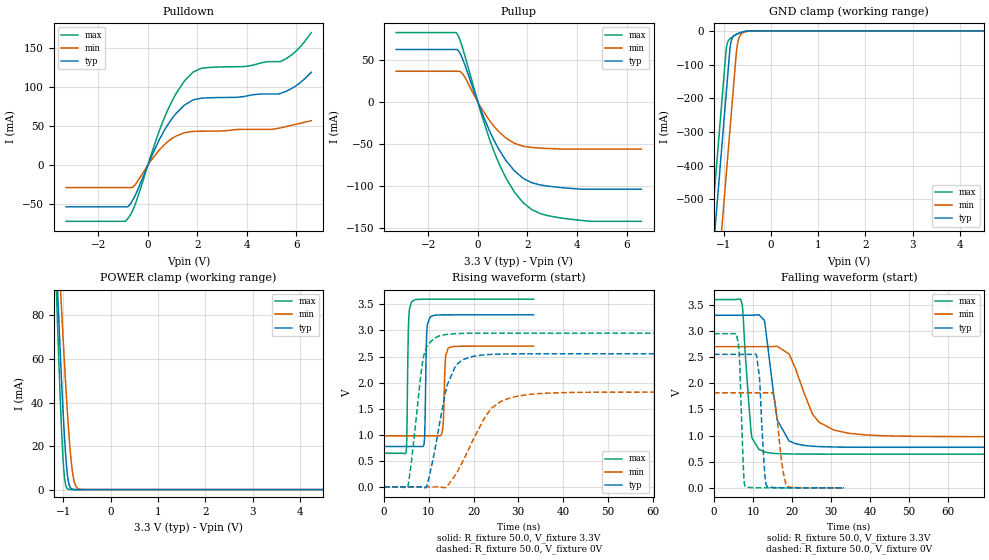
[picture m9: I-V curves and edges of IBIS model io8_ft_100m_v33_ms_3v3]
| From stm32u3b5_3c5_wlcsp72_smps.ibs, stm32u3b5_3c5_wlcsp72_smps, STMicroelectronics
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[Model]   io8_ft_100m_v33_ms_3v3
Model_type I/O
Polarity   Non-Inverting
Enable   Active-Low
| CAP_THRESHOLD on pad IOFT is "UDTCAPC" :
| Rising=30.0% of vddiom   Falling=70.0% of vddiom
| C_comp min and max val. don't necessarily correlate with the min and max pvt
| but are the smallest and greatest pad capacitance found.
| var   typ   min   max
C_comp   5.13864pF  4.98765pF  5.13964pF
|C_comp_pullup   3.32248pF  3.08554pF  3.41453pF
|C_comp_pulldown   1.81616pF  1.90210pF  1.72511pF
Vinl = 1.35V
Vinh = 1.8V
Vmeas = 1.65V   | Reference voltage for timing measurements
Cref  = 50.0pF   | Timing specification test load capacitance value
Rref  = 1.0MOhm   | Timing specification test load resistance value
Vref  = 1.815V   | Timing specification test load voltage
[Model Spec]
| TIME_THRESHOLD on pin ZIV33M is "CMOS" :
| Rising=50.0% of vddiom   Falling=50.0% of vddiom
Vinl 1.27350V 1.06350V 1.35850V
Vinh 1.78850V 1.51250V 1.89250V
| variable   typ   min   max
[Temperature Range] 25.0 130.0 -40.0
| variable   typ   min   max
[Voltage Range] 3.3V 2.7V 3.6V
| variable   typ   min   max
[POWER Clamp Reference] 3.3V 2.7V 3.6V
| variable   typ   min   max
[GND Clamp Reference] 0V 0V 0V
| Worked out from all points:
|   slope of the pulldown table from 0 to 0.495 V, typ, clamps not added: 14.3 ohm
|   slope of the pullup table from 0 to 0.495 V, typ, clamps not added: 13.8 ohm
|   GND clamp passes 1 mA (typ) near -0.50 V on its own axis
|   POWER clamp passes 1 mA (typ) near -0.85 V on its own axis
|   rising waveform, R_fixture 50.0, V_fixture 3.3V: 20-80 % time 305ps typ, 372ps min, 294ps max; typ from 0.776 V to 3.3 V
|   falling waveform, R_fixture 50.0, V_fixture 3.3V: 20-80 % time 2.69ns typ, 5.74ns min, 1.65ns max; typ from 3.3 V to 0.776 V
|   rising waveform, R_fixture 50.0, V_fixture 0V: 20-80 % time 3.67ns typ, 6.72ns min, 2.29ns max; typ from 0 V to 2.55 V
|   falling waveform, R_fixture 50.0, V_fixture 0V: 20-80 % time 1.08ns typ, 1.6ns min, 821ps max; typ from 2.55 V to 0 V
[POWER Clamp]
-3.3V     1.376A     1.183A     1.687A
-1.15V    107mA      132mA      94.23mA
-1.14V    101.7mA    127.5mA    87.74mA
-1.11V    86.11mA    114.3mA    68.77mA
-1.05V    56.42mA    88.49mA    34.19mA
-1V       34.12mA    67.92mA    12.34mA
-960mV    19.14mA    52.36mA    3.231mA
-900mV    4.863mA    31.3mA     221.9uA
-840mV    665uA      14.67mA    12.78uA
-790mV    105.7uA    5.908mA    1.173uA
-650mV    562.2nA    165.6uA    2.035nA
6.6V      0A         0A         0A
[GND Clamp]
-3.3V     -4.192A    -4.434A    -4.059A
-1.25V    -707.2mA   -948.8mA   -574.2mA
-950mV    -197.2mA   -438.8mA   -64.18mA
-940mV    -180.2mA   -421.8mA   -51.24mA
-870mV    -61.19mA   -302.8mA   -24.27mA
-850mV    -38.62mA   -268.8mA   -21.84mA
-800mV    -17.58mA   -183.8mA   -16.98mA
-730mV    -9.777mA   -65.72mA   -11.28mA
-710mV    -8.51mA    -43.04mA   -9.847mA
-620mV    -4.247mA   -8.765mA   -4.565mA
-390mV    -85.77uA   -309.6uA   -31.83uA
6.6V      2.503nA    356.6nA    1.779nA
| variable   typ   min   max
[Pullup Reference] 3.3V 2.7V 3.6V
| variable   typ   min   max
[Pulldown Reference] 0V 0V 0V
[Pullup]
-3.3V     62.95mA    36.94mA    83.15mA
-850mV    62.83mA    36.94mA    82.03mA
-580mV    48.78mA    32.19mA    60.8mA
140mV     -11.12mA   -7.203mA   -14.31mA
460mV     -33.8mA    -21.6mA    -43.61mA
800mV     -53.86mA   -33.82mA   -69.73mA
1.14V     -69.93mA   -42.96mA   -90.97mA
1.48V     -82.17mA   -49.14mA   -107.6mA
2.17V     -96.08mA   -54mA      -128.2mA
2.85V     -100.3mA   -55.28mA   -135.6mA
3.88V     -103.2mA   -56.04mA   -140.2mA
6.6V      -103.8mA   -56.04mA   -142.2mA
[Pulldown]
-3.3V     -53.27mA   -28.52mA   -71.84mA
-850mV    -53.27mA   -28.52mA   -70.02mA
-500mV    -38.18mA   -24.47mA   -49.51mA
460mV     32.61mA    19.53mA    43.99mA
800mV     51.7mA     30.09mA    70.55mA
1.14V     66.56mA    37.47mA    92mA
1.48V     77.24mA    41.82mA    108.3mA
1.83V     83.91mA    43.43mA    119.6mA
2.17V     86.16mA    43.73mA    124.5mA
5.35V     92.17mA    47.94mA    133mA
5.95V     101.3mA    52.36mA    145.4mA
6.6V      119.3mA    57.17mA    170.3mA
[Ramp]
dV/dt_r 1.53142V/3.42869ns 1.09015V/6.61674ns 1.76896V/2.2851ns
dV/dt_f 1.51461V/2.59898ns 1.03189V/5.56958ns 1.77292V/1.6389ns
R_load = 50.0
| Removed startup time: 0s 0s 0s  .
| Removed end time: 33.4ns.
[Rising Waveform]
R_fixture   = 50.0
V_fixture   = 3.3V
V_fixture_min = 2.7V
V_fixture_max = 3.6V
0s        775.7mV    980.2mV    645.1mV
4.95ns    775.7mV    980.2mV    676.5mV
5.5ns     775.7mV    980.2mV    3.146V
6.15ns    775.7mV    980.2mV    3.545V
8.95ns    829.6mV    980.2mV    3.598V
9.55ns    2.945V     980.2mV    3.598V
10.25ns   3.251V     980.2mV    3.598V
12.95ns   3.297V     1.024V     3.599V
14.35ns   3.298V     2.663V     3.6V
33.4ns    3.3V       2.7V       3.6V
| Removed startup time: 0s 0s 0s  .
| Removed end time: 188.4ns.
[Falling Waveform]
R_fixture   = 50.0
V_fixture   = 3.3V
V_fixture_min = 2.7V
V_fixture_max = 3.6V
0s        3.3V       2.7V       3.6V
6.85ns    3.3V       2.7V       3.597V
9.7ns     3.3V       2.7V       971.2mV
12.9ns    3.204V     2.7V       689.8mV
13.85ns   2.667V     2.7V       673.2mV
16.2ns    1.297V     2.706V     655mV
22.95ns   813.3mV    1.846V     646mV
26.9ns    788.9mV    1.257V     645.4mV
38.45ns   776.6mV    1.015V     645.1mV
188.4ns   775.7mV    980.2mV    645.1mV
| Removed startup time: 0s 0s 0s  .
| Removed end time: 98.35ns.
[Rising Waveform]
R_fixture   = 50.0
V_fixture   = 0V
V_fixture_min = 0V
V_fixture_max = 0V
0s        11.93nV    102.1nV    24.43nV
5.3ns     10.58nV    101.6nV    -6.765mV
8.8ns     -9.139mV   105.4nV    2.478V
10.05ns   171.5mV    551.1nV    2.751V
12.05ns   1.032V     99.3uV     2.883V
14.05ns   1.938V     4.493mV    2.924V
16.05ns   2.334V     239.3mV    2.939V
22.7ns    2.534V     1.357V     2.948V
28.1ns    2.549V     1.705V     2.948V
98.35ns   2.552V     1.817V     2.948V
| Removed startup time: 0s 0s 0s  .
| Removed end time: 33.35ns.
[Falling Waveform]
R_fixture   = 50.0
V_fixture   = 0V
V_fixture_min = 0V
V_fixture_max = 0V
0s        2.552V     1.817V     2.948V
6.15ns    2.552V     1.817V     2.789V
7.95ns    2.552V     1.817V     31.46mV
10.9ns    2.527V     1.817V     2.426mV
11.65ns   2.105V     1.817V     1.678mV
13ns      281.9mV    1.817V     964.2uV
13.65ns   25.19mV    1.817V     785uV
15.7ns    4.734mV    1.636V     405uV
18.4ns    1.453mV    75.15mV    180.9uV
33.35ns   51.16uV    474.7uV    2.272uV
